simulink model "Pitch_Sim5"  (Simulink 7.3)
settings: Solver=ode45  StartTime=0.0  StopTime=200  RelTol=1e-3
InitFcn:
  | init
StartFcn:
  | init
StopFcn:
  | pl
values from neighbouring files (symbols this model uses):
  d2r = 1/r2d    (= 0.0174532925199)    [init.m]    (also in freq.m; frequ.m; init_lat.m; pl.m)
undefined symbols (not defined in the file or in its folder): Acl, Bcl, Ccl, Dcl

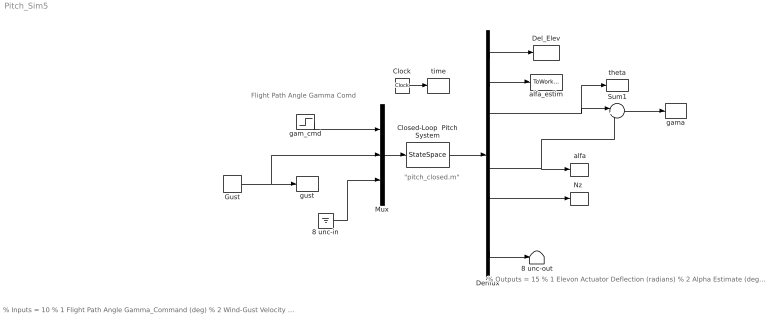
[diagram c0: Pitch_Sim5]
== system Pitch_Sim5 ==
  note: Flight Path Angle Gamma Comd
  note: % Outputs = 15 % 1 Elevon Actuator Deflection (radians) % 2 Alpha Estimate (deg) % 3 Pitch Attitude (thet-123) (radians) % 4 Pitch Rate (q-body) (rad/sec) % 5 Angle of attack, alfa, (radians) % 6 Accelerom # 2, (along Z), (ft/sec^2) Translat. Acceler % 7 Alpha Sensed at Vane # 1 (radian) % 8 Cm_alpha : -36.364 % Variation % 9 Cz_alpha : -21.875 % Variation % 10 Cm_0 : -27.027 % Variation % 11 CZ_0 : -50.000 % Variation % 12 I_yy : 4.232 % Variation % 13 Xcg locat: 1.909 % Variation % 14 Cz_surf 1: -32.184 % Variation % 15 Cm_surf 1: -34.722 % Variation
  note: % Inputs = 10 % 1 Flight Path Angle Gamma_Command (deg) % 2 Wind-Gust Velocity pre-shaped (ft/sec) % 3 Cm_alpha : -36.364 % Variation % 4 Cz_alpha : -21.875 % Variation % 5 Cm_0 : -27.027 % Variation % 6 CZ_0 : -50.000 % Variation % 7 I_yy : 4.232 % Variation % 8 Xcg locat: 1.909 % Variation % 9 Cz_surf 1: -32.184 % Variation % 10 Cm_surf 1: -34.722 % Variation
  note: "pitch_closed.m"
  " alfa" : ToWorkspace  VariableName=alfa  SampleTime=-1  SaveFormat=Array
  8 unc-in : Ground
  8 unc-out : Terminator
  Clock : Clock
  Closed-Loop  Pitch System : StateSpace  A=Acl  B=Bcl  C=Ccl  D=Dcl
  Del_Elev : ToWorkspace  VariableName=delev  SampleTime=-1  SaveFormat=Array
  Demux : Demux  Outputs=[1 1 1 1 1 1 1 8]
  Gust : DiscretePulseGenerator  PulseType=Time based  Amplitude=30  Period=500  PulseWidth=2  PhaseDelay=0  SampleTime=1
  Mux : Mux  Inputs=[1, 1, 8]
  "Nz " : ToWorkspace  VariableName=Nz  SampleTime=-1  SaveFormat=Array
  Sum1 : Sum  Inputs=|+-  OutDataType=fixdt(1, 16)  OutScaling=2^0
  alfa_estim : ToWorkspace  VariableName=alfa_est  SampleTime=-1  SaveFormat=Array
  gam_cmd : Step  After=d2r  SampleTime=0
  gama : ToWorkspace  VariableName=gama  SampleTime=-1  SaveFormat=Array
  gust : ToWorkspace  VariableName=Vgst  SampleTime=-1  SaveFormat=Array
  theta : ToWorkspace  VariableName=theta  SampleTime=-1  SaveFormat=Array
  time : ToWorkspace  VariableName=time  SampleTime=-1  SaveFormat=Array
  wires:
  Closed-Loop  Pitch System/1 -> Demux/1
  Mux/1 -> Closed-Loop  Pitch System/1
  Sum1/1 -> gama/1
  Clock/1 -> time/1
  Demux/1 -> Del_Elev/1
  Demux/2 -> alfa_estim/1
  Demux/3 -> theta/1, Sum1/1
  Demux/5 -> " alfa"/1, Sum1/2
  Demux/6 -> "Nz "/1
  Gust/1 -> gust/1, Mux/2
  gam_cmd/1 -> Mux/1
  8 unc-in/1 -> Mux/3
  Demux/8 -> 8 unc-out/1
